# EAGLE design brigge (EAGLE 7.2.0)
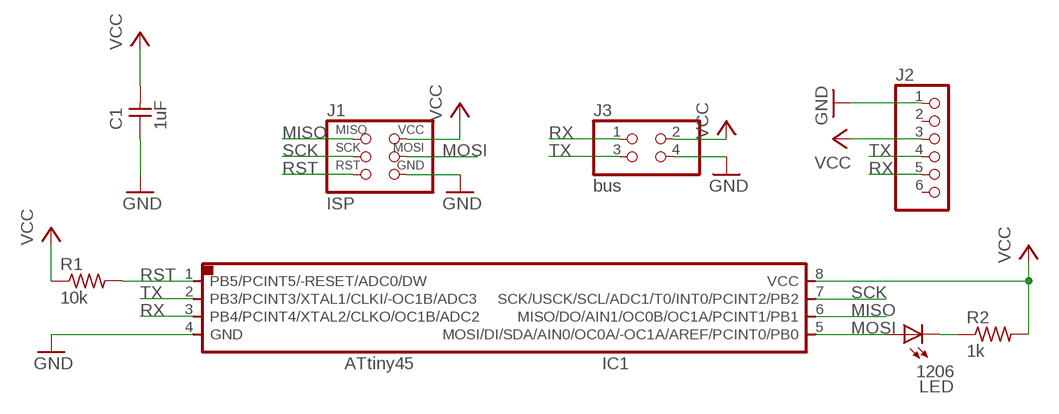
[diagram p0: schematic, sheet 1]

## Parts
C1  1uF  CAP-UNPOLARIZEDFAB  [C1206FAB]
IC1  ATTINY45SI  [SOIC8]
J1  ISP  AVRISPSMD  [2X03SMD]
J2  PINHD-1X6/90  [1X06/90]
J3  bus  PINHD-2X2-SMD  [2X02SMD]
LED  1206  LEDFAB1206  [LED1206FAB]
R1  10k  RES-US1206FAB  [R1206FAB]
R2  1k  RES-US1206FAB  [R1206FAB]

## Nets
GND: C1.1 IC1.4(GND) J1.6(GND) J2.1 J3.4
MISO: IC1.6(MISO/DO/AIN1/OC0B/OC1A/PCINT1/PB1) J1.1(MISO)
MOSI: IC1.5(MOSI/DI/SDA/AIN0/OC0A/-OC1A/AREF/PCINT0/PB0) J1.4(MOSI) LED.1(A)
N$3: LED.2(C) R2.1
RST: IC1.1(PB5/PCINT5/-RESET/ADC0/DW) J1.5(RST) R1.2
RX: IC1.3(PB4/PCINT4/XTAL2/CLKO/OC1B/ADC2) J2.5 J3.1
SCK: IC1.7(SCK/USCK/SCL/ADC1/T0/INT0/PCINT2/PB2) J1.3(SCK)
TX: IC1.2(PB3/PCINT3/XTAL1/CLKI/-OC1B/ADC3) J2.4 J3.3
VCC: C1.2 IC1.8(VCC) J1.2(VCC) J2.3 J3.2 R1.1 R2.2
Unconnected: J2.2 J2.6

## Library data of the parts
C1 = networking:CAP-UNPOLARIZED
IC1 = networking:ATTINY45
J1 = networking:AVRISP
J2 = networking:PINHD-1X6: PIN HEADER
J3 = networking:PINHD-2X2-SMD
LED = networking:LED: LED
R1 R2 = networking:RES-US: Resistor (US Symbol)

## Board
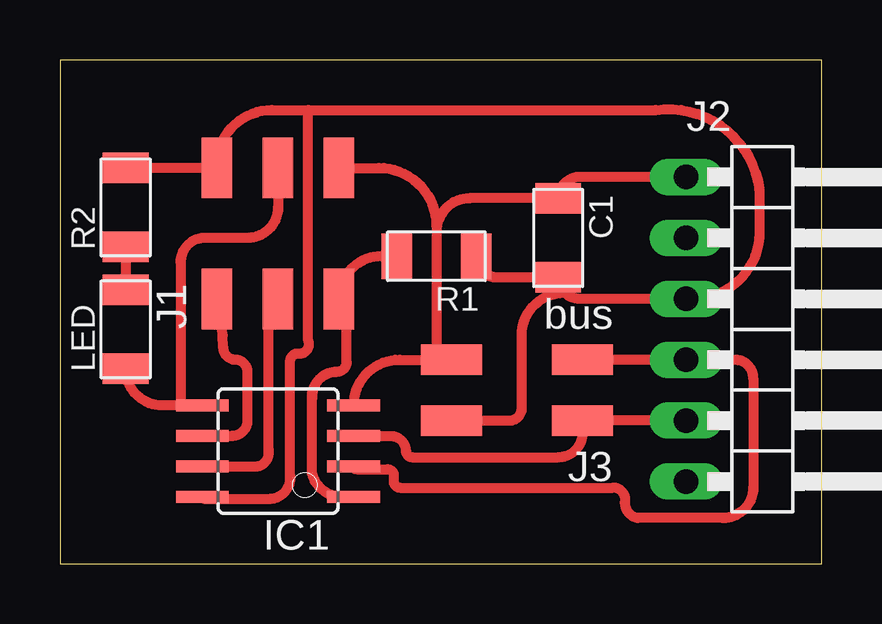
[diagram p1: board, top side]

Size 31.75 x 21 mm. Coordinates in mm from the lower left corner, seen from the top.
Outline: 0,0 31.75,0 31.75,21 0,21 0,0
Copper layers (1*16): Top 0.035mm / dielectric 1.5mm / Bottom 0.035mm
Design rules "default *": minimum track width 10mil, minimum drill 0.6mm, track to track 0.4mm, track to pad 0.4mm, pad to pad 0.4mm, via to via 0.4mm, smd to smd 0.4mm, copper to edge 40mil, drill to drill 8mil, minimum pad ring 10mil, minimum via ring 8mil, stop-mask expansion 4mil, vias tented up to drill 0mil, thermal gap 10mil

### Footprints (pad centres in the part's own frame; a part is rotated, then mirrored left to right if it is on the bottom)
C1206FAB = smd 1.27 x 1.905: 1 -1.651,0; 2 1.651,0
SOIC8 = smd 0.5 x 2.2: 1 -1.905,-3.154; 2 -0.645,-3.154; 3 0.625,-3.154; 4 1.895,-3.154; 5 1.905,3.154; 6 0.635,3.154; 7 -0.635,3.154; 8 -1.905,3.154
2X03SMD = smd 2.54 x 1.27: 1 -2.54,2.54; 2 2.92,2.54; 3 -2.54,0; 4 2.92,0; 5 -2.54,-2.54; 6 2.92,-2.54
1X06/90 = drill 1.016 long: 1 -6.35,-3.81; 2 -3.81,-3.81; 3 -1.27,-3.81; 4 1.27,-3.81; 5 3.81,-3.81; 6 6.35,-3.81
2X02SMD = smd 2.54 x 1.27: 1 -2.54,1.27; 2 2.92,1.27; 3 -2.54,-1.27; 4 2.92,-1.27
LED1206FAB = smd 1.27 x 1.905: 1 -1.651,0; 2 1.651,0
R1206FAB = smd 1.27 x 1.905: 1 -1.651,0; 2 1.651,0

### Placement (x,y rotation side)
C1  20.77,13.58 270 top
IC1  9.09,4.69 90 top
J1  9.09,13.58 90 top
J2  29.92,9.77 270 top
J3  19.25,7.23 180 top
LED  2.74,9.77 90 top
R1  15.69,12.82 180 top
R2  2.74,14.85 90 top

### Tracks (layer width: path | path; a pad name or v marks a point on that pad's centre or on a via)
GND
  Top 0.406: J1.6 13.28,16.5 arc-90 15.69,14.09 | 15.69,14.09 15.69,14.34 | 15.69,14.09 15.69,13.83 | 16.33,8.88 J3.4 15.69,8.5 | J2.1 21.66,16.12 arc90 C1.1 17.09,15.23 arc90 15.69,13.83 | 15.69,13.83 15.69,8.5 | IC1.4 arc-90 14.16,8.5 15.69,8.5
MISO
  Top 0.406: IC1.6 7.18,5.33 arc90 7.82,5.96 7.82,7.99 arc90 7.31,8.5 arc-90 6.8,9.01 arc14 J1.1
MOSI
  Top 0.406: IC1.5 5.03,6.59 | 5.03,6.59 4.26,6.59 arc-90 LED.1 | J1.4 9.09,14.85 arc-90 7.82,13.58 6.04,13.58 arc90 5.03,12.56 5.03,6.59
  Top 0.61: 2.74,7.87 LED.1
N$3
  Top 0.406: R2.1 LED.2
RST
  Top 0.406: IC1.1 arc-90 10.51,3.76 10.51,6.9 10.51,6.96 arc-90 11.55,8 arc90 11.95,8.4 11.95,10.55 arc-90 11.63,10.87 J1.5 | 11.88,10.79 arc90 J1.5 | R1.2 13.41,12.82 arc90 J1.5
RX
  Top 0.406: J2.5 J3.1 21.79,5.45 arc-90 20.77,4.44 14.68,4.44 arc-90 14.42,4.69 arc90 13.8,5.32 IC1.3
SCK
  Top 0.406: IC1.7 8.26,4.05 arc90 8.69,4.74 8.7,4.74 8.7,10.3 9.09,10.3 J1.3
TX
  Top 0.406: J3.3 J2.4 28.14,8.5 arc-90 28.9,7.74 28.9,3.17 arc-90 27.63,1.9 24.08,1.9 arc-90 23.57,2.66 arc90 23.06,3.17 14.17,3.17 arc-90 13.92,3.42 13.92,3.67 arc90 13.66,3.93 12.36,3.93 arc-90 IC1.2
VCC
  Top 0.406: C1.2 arc90 21.66,11.04 J2.3 arc90 29.16,13.58 29.16,15.61 arc90 24.84,18.91 10.35,18.91 | C1.2 18.23,11.93 arc-90 R1.1 | J3.2 18.74,5.96 arc90 19.25,6.47 19.25,9.52 arc-90 21.03,11.29 21.03,11.68 arc90 C1.2 | R2.2 J1.2 arc-90 J1.2 6.55,16.63 arc-90 8.84,18.91 10.35,18.91 | 5.92,2.79 IC1.8 arc90 6.02,2.7 8.8,2.7 arc90 9.6,3.65 9.6,8.5 arc-90 10,8.75 arc108 10.35,9.3 10.35,18.91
